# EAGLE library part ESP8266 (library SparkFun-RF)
Espressif ESP8266 WiFi/Microcontroller SoC The ESP8266 WiFi Module is a self contained SOC with integrated TCP/IP protocol stack that can give any microcontroller access to your WiFi network. The ESP8266 is capable of either hosting an application or offloading all Wi-Fi networking functions from another application processor. SparkFun Products WiFi Module ESP8266 (WRL-13678) SparkFun ESP8266 Thing (WRL-13231) SparkFun WiFi Shield - ESP8266 (WRL-13287) SparkFun ESP8266 Thing - Dev Board (WRL-13711) SparkFun Blynk Board - ESP8266 (WRL-13794)
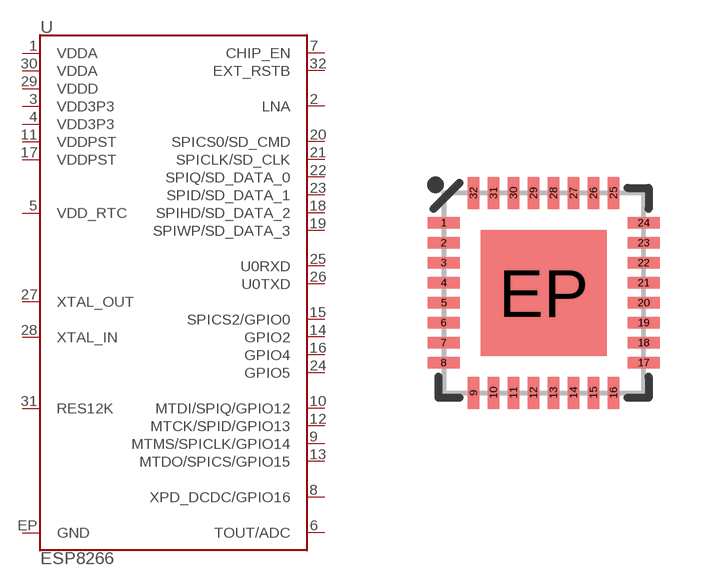
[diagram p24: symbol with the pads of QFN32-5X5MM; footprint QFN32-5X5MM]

Designator prefix U

## ESP8266 (PROD_ID: IC-12452)  [QFN32-5X5MM]
1  VDDA
2  LNA
3  VDD3P3
4  VDD3P3
5  VDD_RTC
6  TOUT/ADC
7  CHIP_EN
8  XPD_DCDC/GPIO16
9  MTMS/SPICLK/GPIO14
10  MTDI/SPIQ/GPIO12
11  VDDPST
12  MTCK/SPID/GPIO13
13  MTDO/SPICS/GPIO15
14  GPIO2
15  SPICS2/GPIO0
16  GPIO4
17  VDDPST
18  SPIHD/SD_DATA_2
19  SPIWP/SD_DATA_3
20  SPICS0/SD_CMD
21  SPICLK/SD_CLK
22  SPIQ/SD_DATA_0
23  SPID/SD_DATA_1
24  GPIO5
25  U0RXD
26  U0TXD
27  XTAL_OUT
28  XTAL_IN
29  VDDD
30  VDDA
31  RES12K
32  EXT_RSTB
EP  GND

## Footprint QFN32-5X5MM (pad centres in mm)
32-pin QFN 5.0 x 5.0 mm, 0.5mm pitch Used by ESP8266 Datasheet
smd 0.8 x 0.285: 1 -2.5,1.75; 2 -2.5,1.25; 3 -2.5,0.75; 4 -2.5,0.25; 5 -2.5,-0.25; 6 -2.5,-0.75; 7 -2.5,-1.25; 8 -2.5,-1.75; 17 2.5,-1.75; 18 2.5,-1.25; 19 2.5,-0.75; 20 2.5,-0.25; 21 2.5,0.25; 22 2.5,0.75; 23 2.5,1.25; 24 2.5,1.75
smd 0.285 x 0.8: 9 -1.75,-2.5; 10 -1.25,-2.5; 11 -0.75,-2.5; 12 -0.25,-2.5; 13 0.25,-2.5; 14 0.75,-2.5; 15 1.25,-2.5; 16 1.75,-2.5; 25 1.75,2.5; 26 1.25,2.5; 27 0.75,2.5; 28 0.25,2.5; 29 -0.25,2.5; 30 -0.75,2.5; 31 -1.25,2.5; 32 -1.75,2.5
smd 3.15 x 3.15: EP 0,0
